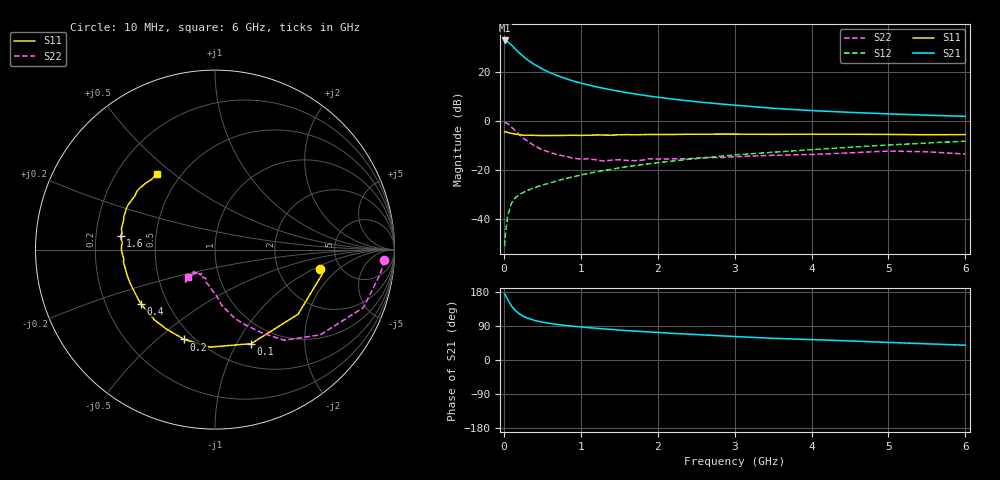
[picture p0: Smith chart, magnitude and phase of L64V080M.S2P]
!  INFINEON TECHNOLOGIES Small Signal Semiconductors
! BFR380L3 , Si-NPN RF-Transistor in TSLP-3-1
!  Vce=4 V,  Ic=80 mA
! Common Emitter S-Parameters:  07. March 2005
#  GHz  S  MA  R  50
! f  S11  S21  S12  S22
! GHz  Mag  Ang  Mag  Ang  Mag  Ang  Mag  Ang
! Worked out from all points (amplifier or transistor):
!   36 points, 10 MHz to 6 GHz, reference 50 ohm
!   highest |S21| = 32.9 dB at 10 MHz (marker M1)
!   |S21| within 3 dB of that: start of sweep to 134.8 MHz
!   unconditionally stable (mu >= 1): 1.25 GHz to 4.837 GHz
!   at 250 MHz: K = 0.53, MSG = 27.8 dB, |S12| = -29.2 dB
!   at 1.4 GHz: K = 1.02, MAG = 15.4 dB, |S12| = -19.7 dB
!   at 6 GHz: K = 0.97, MSG = 5.1 dB, |S12| = -8.2 dB
!   S11 on the Smith chart (normalised r, x): 10 MHz: 3.50, -1.16; 100 MHz: 0.75, -1.15; 200 MHz: 0.44, -0.62; 400 MHz: 0.35, -0.29; 1.6 GHz: 0.31, +0.07; 6 GHz: 0.37, +0.44
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0.01  0.5932 -10.4  44.37 174.1  0.0028 73.5  0.9459 -3.6
0.02  0.6123 -13.1  44.24 171.7  0.0048 81.7  0.9306 -8.4
0.05  0.5862 -37.9  41.75 159.2  0.0118 75.8  0.888 -21.3
0.1  0.5616 -68.9  35.7 142.6  0.0211 64.4  0.7551 -39.0
0.15  0.5441 -92.9  29.7 130.3  0.0275 57.6  0.6356 -52.6
0.2  0.5291 -108.9  24.82 122.0  0.0315 56.4  0.5341 -60.5
0.25  0.5188 -121.2  21.14 115.9  0.0348 53.7  0.4495 -68.3
0.3  0.5169 -130.5  18.2 111.2  0.0384 54.3  0.3989 -73.9
0.4  0.5122 -144.1  14.23 104.4  0.0438 55.0  0.3116 -83.2
0.5  0.5071 -152.7  11.63 100.0  0.0496 57.8  0.2602 -87.8
0.6  0.5084 -159.0  9.751 96.4  0.0547 59.4  0.2302 -93.3
0.7  0.51 -163.6  8.448 93.7  0.061 61.2  0.2059 -98.7
0.9  0.5149 -172.0  6.621 89.1  0.0728 63.9  0.1751 -107.7
1.1  0.5164 -177.1  5.473 85.3  0.0857 65.4  0.1703 -112.7
1.3  0.5209 177.5  4.673 82.0  0.0984 66.5  0.1528 -119.7
1.6  0.5307 171.7  3.814 77.6  0.1172 67.2  0.158 -127.2
2.2  0.534 162.8  2.815 70.3  0.1538 67.5  0.1697 -128.6
2.8  0.545 154.5  2.25 64.1  0.1904 67.4  0.1793 -134.8
3.5  0.5376 146.3  1.831 57.2  0.2315 65.2  0.2009 -133.3
4.5  0.5402 140.2  1.511 50.3  0.2935 63.4  0.225 -132.8
5.5  0.5273 132.2  1.323 42.7  0.3573 59.6  0.2366 -132.6
6  0.5316 127.2  1.254 39.0  0.3907 57.4  0.2129 -134.4
